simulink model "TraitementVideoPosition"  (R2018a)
settings: Solver=ode45  StartTime=0.0  StopTime=inf  RelTol=1e-3  EnableMultiTasking=on
undefined symbols (not defined in the file): adaptor, C, Cinema, f88c69eb4c3a, genericvideo, gray, imaq, intmax, IsPositionTracked, IsSkeletonTracked, JointDepthIndices, JointImageIndices, JointTrackingState, JointWorldCoordinates, LifeCam, lineargauge, MATLAB, Microsoft, none, PositionDepthIndices, PositionImageIndices, PositionWorldCoordinates, ProgramData, R2018a, SegmentationData, SkeletonTrackingID, SuiviBlob, SupportPackages, supportpackages, TM, toolbox, videoinput, win64, winvideo
libraries: simulink x2, dspindex x2, visionstatistics x1, visiontextngfix x1, imaqlib x1

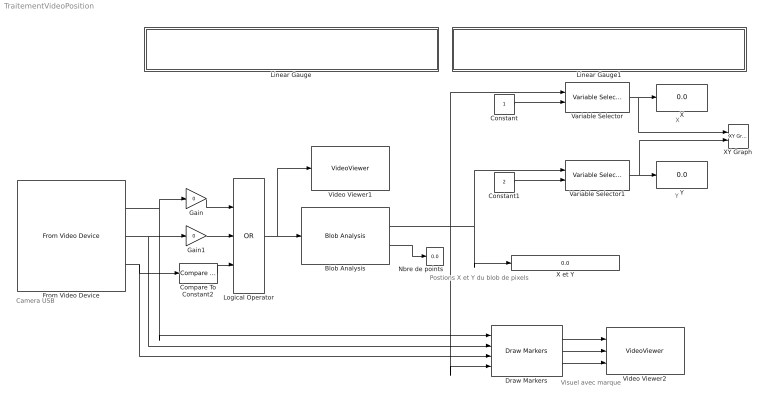
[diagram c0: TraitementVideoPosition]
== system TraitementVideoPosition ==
  note: Camera USB
  note: Visuel avec marque
  note: Postions X et Y du blob de pixels
  note: Y
  note: X
  Blob Analysis : visionstatistics/Blob Analysis  Tag=vipblks_row_conv  area=off  centroid=on  bBox=off  majorAxis=off  minorAxis=off  angle=off  eccentricity=off  equivDiameterSq=off  extent=off  perimeter=off  maxBlobs=1  warnIfNumBlobsExceeded=on  isCount=on  useMinArea=off  minArea=0  useMaxArea=off  maxArea=intmax('uint32')  excludeBorderBlob=off  outDT=double  isOutVarDim=off  isFill=on  fillValues=-1  conn=8  isLabel=off  outputMode=Binary point scaling  outputWordLength=32  outputFracLength=16  firstCoeffMode=Binary point scaling  firstCoeffWordLength=16  firstCoeffFracLength=14  secondCoeffMode=Binary point scaling  secondCoeffWordLength=32  secondCoeffFracLength=16  accumMode=Binary point scaling  accumWordLength=32  accumFracLength=0  prodOutputMode=Binary point scaling  prodOutputWordLength=32  prodOutputFracLength=16  roundingMode=Floor  overflowMode=off
  Compare To Constant2 : simulink/Logic and Bit Operations/Compare To Constant  relop=>=  const=0.97  OutDataTypeStr=boolean
  Constant : Constant
  Constant1 : Constant  Value=2
  Draw Markers : visiontextngfix/Draw Markers  shape=X-mark  size=5  fill=off  fillClrSource=Specify via dialog  display=Black  intensity=200  color=[200 255 100]  opacity=0.6  viewport=Entire image  antialiasing=off  inType=Obsolete  imagePorts=Separate color signals  prodOutputMode=Binary point scaling  prodOutputWordLength=32  prodOutputFracLength=14  memoryMode=Specify word length  memoryWordLength=16  memoryFracLength=15  roundingMode=Floor  overflowMode=off
  From Video Device : imaqlib/From Video Device  DeviceMenu=(none)  Device=winvideo 1 (Microsoft® LifeCam Cinema(TM))  ObjConstructor=videoinput('winvideo', 1)  VideoFormatMenu=(none)  VideoFormat=YUY2_640x360  VideoSource=input1  ROIPosition=[0 0 360 640]  EnableHWTrigger=off  TriggerConfiguration=none/none  SampleTime=1/30  OutputPortsMode=Separate color signals  DataType=single  CanDoHWTrigger=no  ReturnedColorSpace=rgb  BlockHandle=1921.0006  ROIWidth=640  ROIHeight=360  ROIColumn=0  ROIRow=0  EngXMLPath=C:\Program Files\MATLAB\R2018a\toolbox\imaq\imaq\private  DevXMLPath=C:\ProgramData\MATLAB\SupportPackages\R2018a\toolbox\imaq\supportpackages\genericvideo\adaptor\win64  EngLibPath=C:\Program Files\MATLAB\R2018a\toolbox\imaq\imaqblks\imaqmex\win64  ColorSpace=rgb  BayerSensorAlignment=grbg  AllMetadata=IsPositionTracked;IsSkeletonTracked;JointDepthIndices;JointImageIndices;JointTrackingState;JointWorldCoordinates;PositionDepthIndices;PositionImageIndices;PositionWorldCoordinates;SegmentationData;SkeletonTrackingID
  Gain : Gain  Gain=0
  Gain1 : Gain  Gain=0
  Linear Gauge : Subsystem  DialogController=hmiCreateDDGDialog  IsWebBlock=on  mask(MWDashboardBlock){webBlockId=382084fc-5131-4d1a-87ef-f88c69eb4c3a, webBlockType=lineargauge, ShowInLibBrowser=on, ShowInitialText=on, HMISrcModelName=SuiviBlob}
      mask prompts: webBlockId "WebBlock Id"; webBlockType "WebBlock Type"; HMISrcModelName "Source Model"
      mask help: SimulinkHMI:dialogs:LinearGaugeDialogDesc
  Linear Gauge1 : Subsystem  DialogController=hmiCreateDDGDialog  IsWebBlock=on  mask(MWDashboardBlock){webBlockId=0c4e6124-9b84-4e5d-82f3-78f2fceaf7e5, webBlockType=lineargauge, ShowInLibBrowser=on, ShowInitialText=on, HMISrcModelName=SuiviBlob}
      mask prompts: webBlockId "WebBlock Id"; webBlockType "WebBlock Type"; HMISrcModelName "Source Model"
      mask help: SimulinkHMI:dialogs:LinearGaugeDialogDesc
  Logical Operator : Logic  Operator=OR  Inputs=3  AllPortsSameDT=off  OutDataTypeStr=boolean
  Nbre de points : Display
  Variable Selector : dspindex/Variable Selector  NumInputs=1  rowsOrCols=Columns  IdxMode=Variable  Elements=[1 3]  ZerOneIdxMode=One-based  errmode=Clip Index  FillMode=on  FillValues=1
  Variable Selector1 : dspindex/Variable Selector  NumInputs=1  rowsOrCols=Columns  IdxMode=Variable  Elements=[1 3]  ZerOneIdxMode=One-based  errmode=Clip Index  FillMode=on  FillValues=1
  Video Viewer1 : VideoViewer  colormapValue=gray(256)  FigPos=[47.6666666666667 742.666666666667 936 624]
  Video Viewer2 : VideoViewer  imagePorts=separate color signals  colormapValue=gray(256)  FigPos=[45.6666666666667 658.666666666667 436 242.666666666667]
  X : Display
  X et Y : Display
  XY Graph : simulink/Sinks/XY Graph  xmin=0  xmax=640  ymin=0  ymax=360  st=-1
  Y : Display
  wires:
  Gain/1 -> Logical Operator/1
  From Video Device/1 -> Gain/1, Draw Markers/1
  From Video Device/2 -> Draw Markers/2, Gain1/1
  Compare To Constant2/1 -> Logical Operator/3
  From Video Device/3 -> Draw Markers/3, Compare To Constant2/1
  Logical Operator/1 -> Blob Analysis/1, Video Viewer1/1
  Blob Analysis/2 -> Nbre de points/1
  Draw Markers/1 -> Video Viewer2/1
  Draw Markers/2 -> Video Viewer2/2
  Draw Markers/3 -> Video Viewer2/3
  Blob Analysis/1 -> Draw Markers/4, X et Y/1, Variable Selector1/1, Variable Selector/1
  Constant/1 -> Variable Selector/2
  Constant1/1 -> Variable Selector1/2
  Variable Selector/1 -> X/1, XY Graph/1
  Variable Selector1/1 -> XY Graph/2, Y/1
  Gain1/1 -> Logical Operator/2

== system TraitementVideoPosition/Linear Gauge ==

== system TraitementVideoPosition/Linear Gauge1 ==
